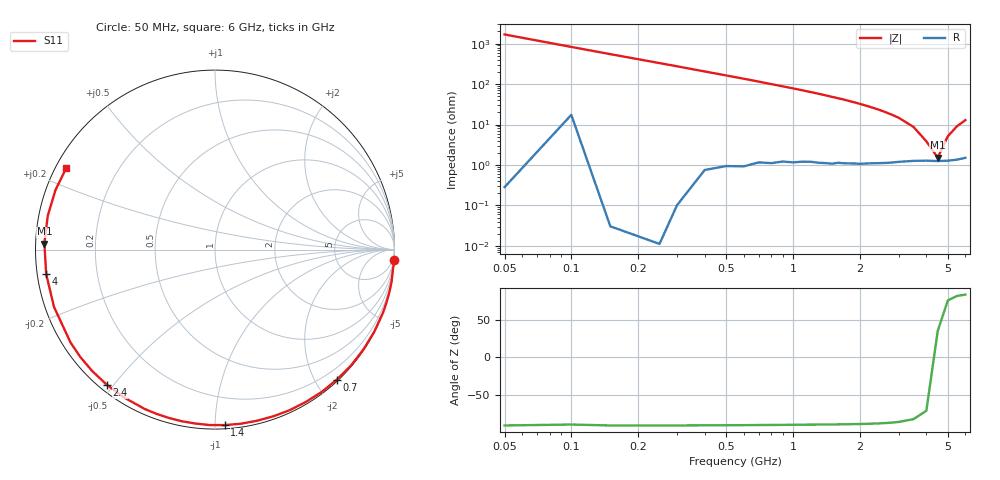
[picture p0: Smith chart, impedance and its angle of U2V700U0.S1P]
! SIEMENS Discrete & RF Semiconductors
! BBY52-02W
! Si Tuning Diode in SCD-80
! VR = 0.7 V
! S-Parameters:  September  1997
# GHz  S  MA  R  50
!  f  S11
! GHz  MAG  ANG
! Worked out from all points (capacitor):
!   34 points, 50 MHz to 6 GHz, reference 50 ohm
!   read as one part to ground: C = 1.92 pF near 50 MHz
!   lowest |Z| = 1.52 ohm at 4.5 GHz (marker M1)
!   series resonance near 4.403 GHz, so ESL is about 680 pH
!   S11 on the Smith chart (normalised r, x): 50 MHz: 0, -34; 700 MHz: 0.02, -2.31; 1.4 GHz: 0.02, -1.06; 2.4 GHz: 0.02, -0.48; 4 GHz: 0.03, -0.07; 6 GHz: 0.03, +0.26
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0.05  1 -3.4
0.2  1 -13.8
0.3  0.9999 -20.6
0.4  0.9983 -27.4
0.5  0.9968 -34.0
0.6  0.9956 -40.5
0.7  0.9927 -46.9
0.8  0.9911 -53.2
0.9  0.9881 -59.3
1  0.9867 -65.1
1.1  0.984 -70.7
1.2  0.9818 -76.3
1.3  0.9808 -81.6
1.4  0.9791 -86.8
1.6  0.975 -96.5
1.8  0.9726 -105.5
2  0.9705 -113.8
2.2  0.9671 -121.6
2.4  0.9646 -128.7
2.6  0.9623 -135.4
2.8  0.9598 -141.6
3  0.9569 -147.3
3.5  0.9521 -160.4
4  0.9504 -171.7
4.5  0.9513 178.0
5  0.9506 168.6
5.5  0.9488 159.6
6  0.9451 151.3
